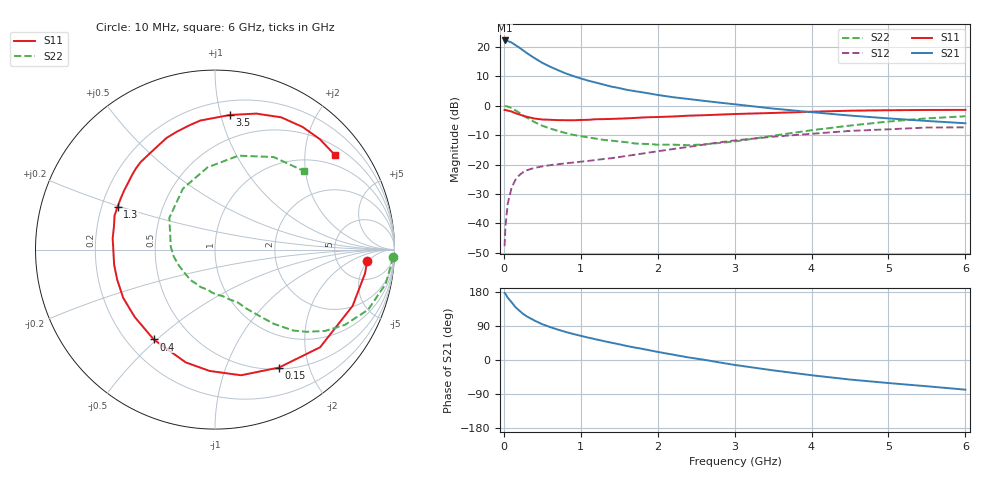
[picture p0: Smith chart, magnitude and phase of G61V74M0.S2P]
! SIEMENS Small Signal Semiconductors
! BFG193
! Si NPN RF Bipolar Junction Transistor in SOT223
! VCE = 1.75 V  IC = 4 mA
! Common Emitter S-Parameters:  August  1996
# GHz  S  MA  R  50
!  f  S11  S21  S12  S22
! GHz  MAG  ANG  MAG  ANG  MAG  ANG  MAG  ANG
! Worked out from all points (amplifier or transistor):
!   36 points, 10 MHz to 6 GHz, reference 50 ohm
!   highest |S21| = 22.2 dB at 10 MHz (marker M1)
!   |S21| within 3 dB of that: start of sweep to 230.9 MHz
!   unconditionally stable (mu >= 1): 1.203 GHz to 2.742 GHz
!   at 250 MHz: K = 0.29, MSG = 20.7 dB, |S12| = -22.6 dB
!   at 1.4 GHz: K = 1.09, MAG = 10.3 dB, |S12| = -17.8 dB
!   at 6 GHz: K = 0.94, MSG = 0.7 dB, |S12| = -7.3 dB
!   S11 on the Smith chart (normalised r, x): 10 MHz: 10, -5; 150 MHz: 0.52, -1.55; 400 MHz: 0.31, -0.49; 1.3 GHz: 0.27, +0.20; 3.5 GHz: 0.31, +1.07; 6 GHz: 0.72, +2.73
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0.01  0.8501 -4.4  12.9 176.9  0.0041 90.8  0.9899 -2.3
0.02  0.8464 -9.0  12.86 174.8  0.0086 84.6  0.9859 -4.6
0.05  0.8286 -22.2  12.63 164.7  0.0215 77.6  0.9702 -11.3
0.1  0.7994 -42.9  11.88 152.7  0.04 68.8  0.9169 -21.4
0.15  0.7477 -61.5  10.76 139.7  0.0548 59.0  0.8363 -30.1
0.2  0.715 -78.3  9.78 130.5  0.0658 52.5  0.7621 -36.5
0.25  0.6767 -92.6  8.751 121.8  0.0742 47.0  0.6856 -41.9
0.3  0.6491 -104.6  7.853 114.9  0.0801 43.0  0.6283 -45.9
0.4  0.606 -124.3  6.45 104.0  0.088 37.4  0.5277 -51.6
0.5  0.584 -140.0  5.369 94.4  0.0931 33.6  0.4574 -55.4
0.6  0.578 -152.2  4.632 87.0  0.0977 31.9  0.4111 -58.6
0.7  0.5701 -163.0  4.049 80.3  0.1011 30.9  0.3759 -61.6
0.9  0.5663 -179.6  3.21 68.8  0.1084 30.3  0.3212 -66.6
1.1  0.5773 167.3  2.666 59.0  0.1155 30.8  0.2892 -73.7
1.3  0.5927 156.3  2.283 49.9  0.1245 31.2  0.2628 -80.5
1.6  0.6114 142.0  1.865 36.9  0.1406 30.9  0.2395 -94.3
2.2  0.6568 119.9  1.398 14.1  0.1839 27.6  0.2178 -128.7
2.8  0.7068 101.7  1.132 -6.3  0.2382 19.5  0.233 -170.4
3.5  0.7549 83.6  0.896 -27.3  0.2981 4.7  0.3099 145.2
4.5  0.8241 63.4  0.681 -51.6  0.374 -15.8  0.4605 95.1
5.5  0.8484 46.5  0.552 -69.3  0.4267 -41.1  0.6104 57.7
6  0.8512 38.1  0.504 -78.3  0.4294 -55.3  0.6624 41.2
